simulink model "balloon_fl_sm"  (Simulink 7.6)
settings: Solver=ode45  StartTime=0.0  StopTime=50000  RelTol=1e-3
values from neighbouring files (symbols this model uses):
  C = V*rho_a*c_a    [balloon_init.m]
  f = f / 10    [balloon_init.m]
  g = 9.80665    [balloon_init.m]
  m = input('Inserire le prime due cifre (esclusi zeri) del proprio numero di matricola:\n\n')    [balloon_init.m]
  rho_a = 1.2928    [balloon_init.m]
  Ta = 20+273.15    (= 293.15)    [balloon_init.m]
  theta_t = theta_t/50    [balloon_init.m]
  V = V*m*2    [balloon_init.m]
  x1_0 = x1_d    [balloon_init.m]
  x2_0 = 100    [balloon_init.m]
  x2_d = 120    [balloon_init.m]
  x3_0 = 0    [balloon_init.m]
undefined symbols (not defined in the file or in its folder): Ksmc, lambda
libraries: simulink x2

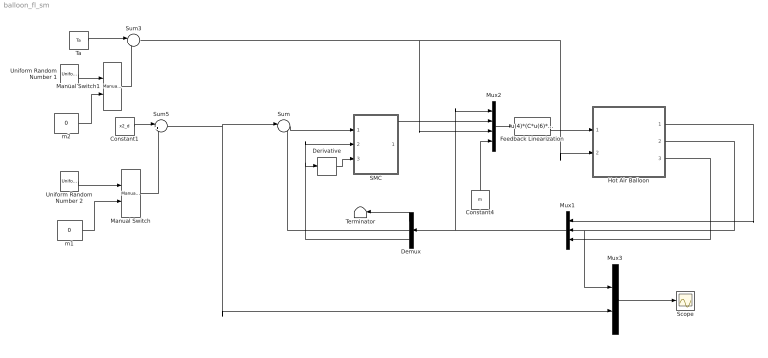
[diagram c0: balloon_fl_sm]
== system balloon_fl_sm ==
  Constant1 : Constant  Value=x2_d
  Constant4 : Constant  Value=m
  Demux : Demux  Outputs=3
  Derivative : Derivative
  Feedback Linearization : Fcn  Expr=u(4)*(C*u(6)*u(1)^2)/(g*V*u(5)*rho_a)-(C*f*u(1))/u(6)+(C*f*u(1)^2)/(u(6)*u(5))-u(5)/theta_t+u(1)/theta_t-(C*f*u(1)^2)/(V*u(5)*rho_a)-(C*f^2+u(1)^2*u(3))/(g*u(6)*V*u(5)*rho_a)
  Hot Air Balloon : Subsystem  mask{V=V, m=m, C=C, theta_t=theta_t, f=f, g=g}
      mask prompts: V "Balloon's volume (V)"; m "Balloon's total mass (m)"; C "Thermal capacitance (C)"; theta_t "Thermal resistance (theta_t)"; f "Aerodynamic viscous friction (f)"; g "Gravitational acceleration (g)"
  Manual Switch : simulink/Signal Routing/Manual Switch  SystemSampleTime=-1  sw=1  action=0  varsize=off
  Manual Switch1 : simulink/Signal Routing/Manual Switch  SystemSampleTime=-1  sw=0  action=0  varsize=off
  Mux1 : Mux  Inputs=3
  Mux2 : Mux
  Mux3 : Mux  Inputs=2
  SMC : Subsystem
  Scope : Scope
  Sum : Sum  Inputs=|-+
  Sum3 : Sum  Inputs=|++
  Sum5 : Sum  Inputs=|++
  Ta : Constant  Value=Ta
  Terminator : Terminator
  Uniform Random Number 1 : UniformRandomNumber  SampleTime=200
  Uniform Random Number 2 : UniformRandomNumber  Minimum=-x2_d*0.1  Maximum=x2_d*0.1  Seed=1  SampleTime=1500
  m1 : Constant  Value=0
  m2 : Constant  Value=0
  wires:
  Hot Air Balloon/3(x3) -> Mux1/3
  Hot Air Balloon/2(x2) -> Mux1/2, Mux3/1
  Hot Air Balloon/1(x1) -> Mux1/1
  Ta/1 -> Sum3/1
  Constant1/1 -> Sum5/1
  Sum3/1 -> Hot Air Balloon/2(Ta), Mux2/3
  Uniform Random Number 2/1 -> Manual Switch/1
  Manual Switch/1 -> Sum5/2
  m1/1 -> Manual Switch/2
  m2/1 -> Manual Switch1/2
  Manual Switch1/1 -> Sum3/2
  Uniform Random Number 1/1 -> Manual Switch1/1
  Feedback Linearization/1 -> Hot Air Balloon/1(u)
  SMC/1(Out) -> Mux2/2
  Mux1/1 -> Demux/1, Mux2/1
  Mux2/1 -> Feedback Linearization/1
  Demux/2 -> Sum/2
  Sum/1 -> SMC/1(y)
  Demux/3 -> SMC/2(ydot), Derivative/1
  Derivative/1 -> SMC/3(yddot)
  Demux/1 -> Terminator/1
  Sum5/1 -> Sum/1, Mux3/2
  Constant4/1 -> Mux2/4
  Mux3/1 -> Scope/1

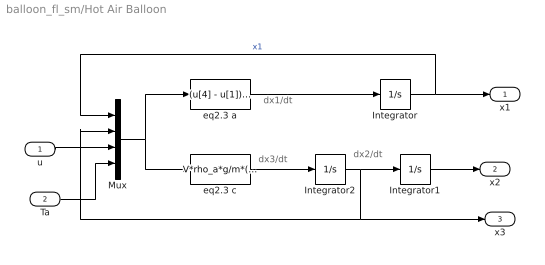
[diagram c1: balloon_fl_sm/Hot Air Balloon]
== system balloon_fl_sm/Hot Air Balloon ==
  note: dx2/dt
  note: dx3/dt
  note: dx1/dt
  u : Inport
  Ta : Inport  Port=2
  Integrator : Integrator  InitialCondition=x1_0
  Integrator1 : Integrator  InitialCondition=x2_0  LowerSaturationLimit=0
  Integrator2 : Integrator  InitialCondition=x3_0
  Mux : Mux
  eq2.3 a : Fcn  Expr=(u[4] - u[1])/(C*theta_t) + u[3]/C
  eq2.3 c : Fcn  Expr=V*rho_a*g/m*(1 - u[4]/u[1]) - f/m*u[2] - g
  x1 : Outport
  x2 : Outport  Port=2
  x3 : Outport  Port=3
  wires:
  Ta/1 -> Mux/4
  u/1 -> Mux/3
  Integrator1/1 -> x2/1
  Integrator2/1 -> Mux/2, x3/1, Integrator1/1
  Integrator/1 -> x1/1, Mux/1  "x1"
  Mux/1 -> eq2.3 c/1, eq2.3 a/1
  eq2.3 c/1 -> Integrator2/1
  eq2.3 a/1 -> Integrator/1

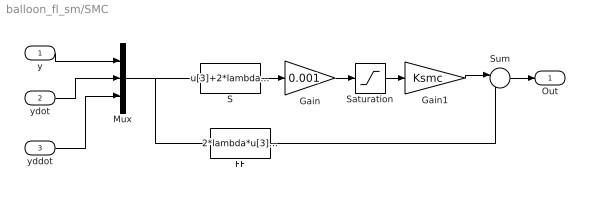
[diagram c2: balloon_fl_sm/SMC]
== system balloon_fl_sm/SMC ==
  y : Inport
  ydot : Inport  Port=2
  yddot : Inport  Port=3
  FF : Fcn  Expr=2*lambda*u[3]+lambda^2*u[2]
  Gain : Gain  Gain=0.001
  Gain1 : Gain  Gain=Ksmc
  Mux : Mux  Inputs=3
  S : Fcn  Expr=u[3]+2*lambda*u[2]+lambda^2*u[1]
  Saturation : Saturate  UpperLimit=1  LowerLimit=-1
  Sum : Sum  Inputs=|--
  Out : Outport
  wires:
  Mux/1 -> FF/1, S/1
  yddot/1 -> Mux/3
  ydot/1 -> Mux/2
  y/1 -> Mux/1
  Sum/1 -> Out/1
  FF/1 -> Sum/2
  Gain1/1 -> Sum/1
  Saturation/1 -> Gain1/1
  Gain/1 -> Saturation/1
  S/1 -> Gain/1
